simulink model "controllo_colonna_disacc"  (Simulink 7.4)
settings: Solver=ode45  StartTime=0.0  StopTime=30.0  RelTol=1e-5
libraries: cstblocks x3

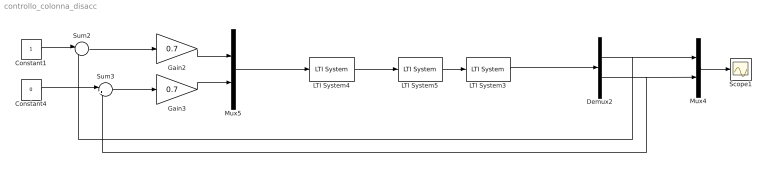
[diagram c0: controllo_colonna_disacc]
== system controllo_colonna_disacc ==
  Constant1 : Constant  OutDataType=sfix(16)  OutScaling=2^0
  Constant4 : Constant  Value=0  OutDataType=sfix(16)  OutScaling=2^0
  Demux2 : Demux  Outputs=2
  Gain2 : Gain  Gain=0.7  ParameterDataType=fixdt(1, 16)  ParameterScaling=2^0  OutDataType=fixdt(1, 16)  OutScaling=2^0
  Gain3 : Gain  Gain=0.7  ParameterDataType=fixdt(1, 16)  ParameterScaling=2^0  OutDataType=fixdt(1, 16)  OutScaling=2^0
  LTI System3 : cstblocks/LTI System  SystemSampleTime=-1  sys=G  IC=[]
  LTI System4 : cstblocks/LTI System  SystemSampleTime=-1  sys=Comp  IC=[]
  LTI System5 : cstblocks/LTI System  SystemSampleTime=-1  sys=L  IC=[]
  Mux4 : Mux  Inputs=2
  Mux5 : Mux  Inputs=2
  Scope1 : Scope
  Sum2 : Sum  Inputs=|+-  OutDataType=sfix(16)  OutScaling=2^0
  Sum3 : Sum  Inputs=|+-  OutDataType=sfix(16)  OutScaling=2^0
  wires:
  Mux4/1 -> Scope1/1
  Demux2/1 -> Sum2/2, Mux4/1
  Demux2/2 -> Mux4/2, Sum3/2
  Gain2/1 -> Mux5/1
  Gain3/1 -> Mux5/2
  Sum2/1 -> Gain2/1
  Sum3/1 -> Gain3/1
  Constant1/1 -> Sum2/1
  Constant4/1 -> Sum3/1
  LTI System3/1 -> Demux2/1
  Mux5/1 -> LTI System4/1
  LTI System5/1 -> LTI System3/1
  LTI System4/1 -> LTI System5/1
